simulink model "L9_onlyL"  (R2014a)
settings: Solver=ode45  StartTime=0.0  StopTime=tend  RelTol=1e-3
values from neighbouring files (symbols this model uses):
  A = [0 1; 0 0]    [L9.m]    (also in L9_LandObs_script.m; L9_fullExample_script.m; L9_onlyL_script.m)
  B = [0; 1]    [L9.m]    (also in L9_LandObs_script.m; L9_fullExample_script.m; L9_onlyL_script.m)
  Cx = eye(size(A))    [L9.m]    (also in L9_LandObs_script.m; L9_fullExample_script.m; L9_onlyL_script.m)
  Dx = zeros(size(Cx,1),size(B,2))    [L9.m]    (also in L9_LandObs_script.m; L9_fullExample_script.m; L9_onlyL_script.m)
  h = h3    (= 0.5)    [L9.m]    (also in L9_LandObs_script.m = 0.44; L9_fullExample_script.m = 0.44; L9_onlyL_script.m = 0.44)
  L = L3    [L9.m]    (also in L9_LandObs_script.m = place(Phi,Gamma,pd); L9_fullExample_script.m = place(Phi,Gamma,pd); L9_onlyL_script.m = place(Phi,Gamma,pd))
  x0 = [1;1]    [L9.m]    (also in L9_LandObs_script.m; L9_fullExample_script.m; L9_onlyL_script.m)

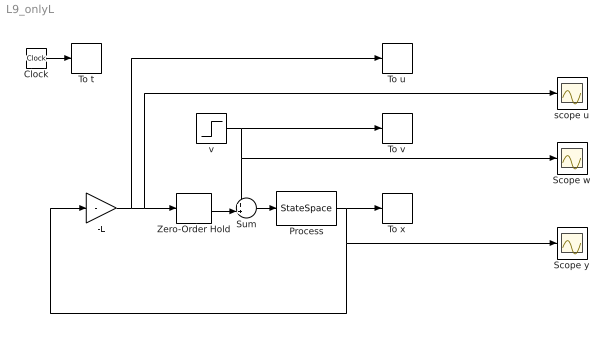
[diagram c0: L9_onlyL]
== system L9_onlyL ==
  -L : Gain  Gain=-L  Multiplication=Matrix(K*u)  SampleTime=h
  Clock : Clock
  Process : StateSpace  A=A  B=B  C=Cx  D=Dx  X0=x0
  Scope w : Scope
  Scope y : Scope
  Sum : Sum  Inputs=++|
  To t : ToWorkspace  VariableName=t  SampleTime=h
  To u : ToWorkspace  VariableName=u  SampleTime=h
  To v : ToWorkspace  VariableName=v  SaveFormat=Structure With Time  SampleTime=-1
  To x : ToWorkspace  VariableName=x  SaveFormat=Structure With Time  SampleTime=-1
  Zero-Order Hold : ZeroOrderHold  SampleTime=h
  scope u : Scope
  v : Step  Time=25  After=-0.5  SampleTime=0
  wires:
  -L/1 -> To u/1, scope u/1, Zero-Order Hold/1
  Clock/1 -> To t/1
  Process/1 -> -L/1, Scope y/1, To x/1
  Sum/1 -> Process/1
  Zero-Order Hold/1 -> Sum/2
  v/1 -> Sum/1, Scope w/1, To v/1
